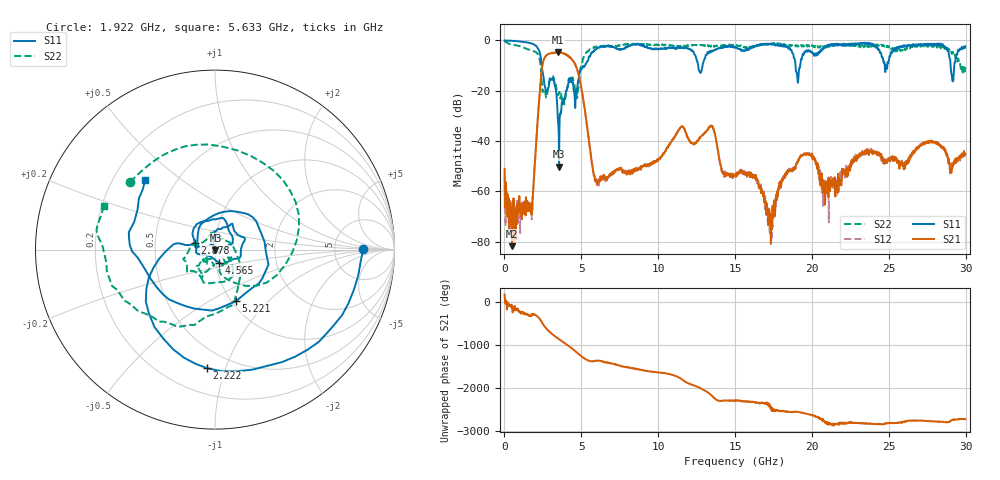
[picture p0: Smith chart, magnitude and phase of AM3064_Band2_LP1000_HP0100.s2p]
# Hz S DB R 50.0
!freq dBS11 angS11 dBS21 angS21 dBS12 angS12 dBS22 angS22
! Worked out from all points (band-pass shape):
!   1600 points, 10 MHz to 29.98 GHz, reference 50 ohm
!   highest |S21| = -4.64 dB at 3.459 GHz (marker M1); lowest = -81.8 dB at 497.3 MHz (marker M2)
!   |S21| within 3 dB of the highest: 2.558 GHz to 4.399 GHz (1.841 GHz wide, 52.9 % of centre)
!   lowest |S11| = -50.1 dB at 3.553 GHz (marker M3), VSWR 1.01, Z = 50.3 - j0.153 ohm
!   |S11| at or under -10 dB: 2.428 GHz to 5.242 GHz (2.814 GHz wide, 73.4 % of centre); 12.6 GHz to 12.88 GHz (283.7 MHz wide, 2.23 % of centre); 18.93 GHz to 19.23 GHz (300.8 MHz wide, 1.58 % of centre)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
!   |S22| runs from -25.4 to -0.2 dB; largest |S21 - S12| = 0.015
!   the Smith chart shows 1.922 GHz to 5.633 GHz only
!   S11 on the Smith chart (normalised r, x): 1.922 GHz: 10, +0; 2.222 GHz: 0.37, -0.86; 2.878 GHz: 0.80, +0.06; 4.565 GHz: 1.04, -0.16; 5.221 GHz: 1.05, -0.67; 5.633 GHz: 0.34, +0.37
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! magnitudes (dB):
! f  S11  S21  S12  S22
! 10 MHz  0.0  -51.0  -53.6  -0.2
! 497.3 MHz  -0.1  -81.8  -67.9  -1.6
! 1.659 GHz  -1.0  -65.9  -64.8  -3.9
! 1.922 GHz  -1.7  -54.9  -53.8  -4.4
! 2.222 GHz  -3.6  -26.5  -26.3  -5.9
! 2.878 GHz  -18.5  -5.3  -5.3  -17.6
! 3.459 GHz  -29.7  -4.6  -4.7  -21.2
! 3.553 GHz  -50.1  -4.9  -4.8  -20.9
! 4.565 GHz  -22.1  -9.1  -9.0  -18.4
! 5.015 GHz  -11.2  -19.3  -19.3  -9.7
! 5.221 GHz  -10.2  -27.2  -27.2  -5.9
! 5.633 GHz  -5.2  -46.5  -46.2  -3.6
! 6.045 GHz  -3.1  -56.0  -56.0  -2.5
! 10 GHz  -3.4  -47.0  -47.3  -1.8
! 13.43 GHz  -4.5  -33.9  -33.9  -2.4
! 15 GHz  -2.5  -53.8  -53.7  -1.8
! 16.37 GHz  -2.0  -54.4  -54.4  -2.3
! 17.25 GHz  -1.4  -71.7  -76.9  -1.2
! 19.99 GHz  -4.5  -46.2  -46.1  -1.9
! 20.95 GHz  -2.6  -58.2  -56.1  -2.2
! 25 GHz  -8.2  -47.5  -46.8  -2.3
! 29.98 GHz  -2.3  -45.1  -45.9  -10.6
